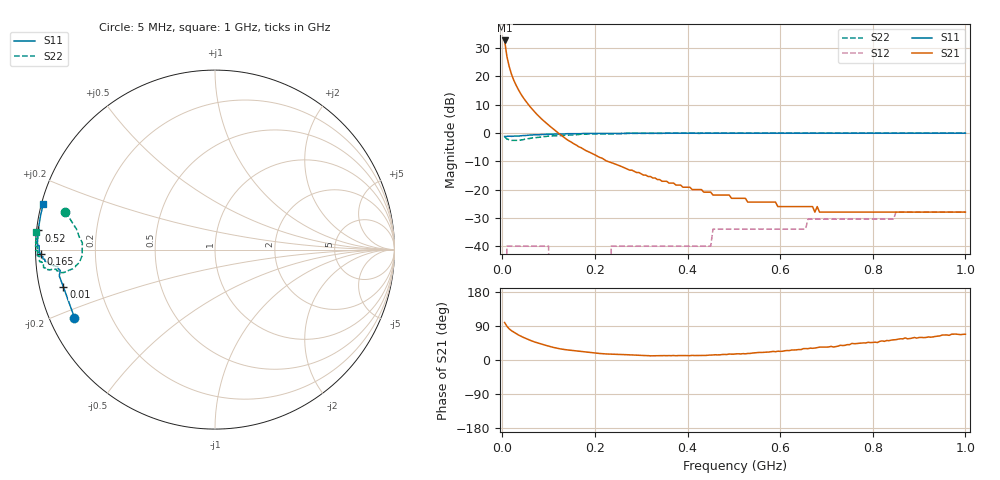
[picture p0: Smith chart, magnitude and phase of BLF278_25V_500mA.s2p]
! Filename:  BLF278_25V_500mA.s2p
! Philips part #: BLF278  !date: 22-05-2003
!Vdd=25V ; Idq=500mA
!D:\Vee measurements\measurement data\VDMOST\BLF278\25V_500mA_#1
# HZ S MA R 50
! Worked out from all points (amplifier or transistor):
!   200 points, 5 MHz to 1 GHz, reference 50 ohm
!   highest |S21| = 32.7 dB at 5 MHz (marker M1)
!   |S21| within 3 dB of that: start of sweep to 7.625 MHz
!   S11 on the Smith chart (normalised r, x): 5 MHz: 0.07, -0.23; 10 MHz: 0.07, -0.12; 165 MHz: 0.02, -0.01; 520 MHz: 0.01, +0.05; 1 GHz: 0.01, +0.13
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5000000  0.87 -154.2  43.03 98.9  0 -7.8  0.86 165.8
1e7  0.87 -166.2  22.29 88.9  0.01 18.0  0.78 171.6
1.5e7  0.88 -170.4  14.8 82.1  0.01 20.1  0.76 174.6
2e7  0.87 -172.3  10.8 77.2  0.01 16.7  0.74 177.1
2.5e7  0.88 -173.1  8.46 73.5  0.01 12.1  0.74 179.5
3e7  0.88 -173.5  6.93 69.6  0.01 6.7  0.74 -179.1
4e7  0.89 -174.0  4.9 62.9  0.01 -1.0  0.75 -175.9
5e7  0.9 -174.3  3.71 57.3  0.01 -7.2  0.78 -173.4
6e7  0.92 -174.7  2.91 52.1  0.01 -12.2  0.8 -172.3
8e7  0.93 -175.5  1.93 43.7  0.01 -18.0  0.84 -171.5
1e8  0.95 -176.3  1.38 36.6  0.01 -18.4  0.88 -171.8
1.05e8  0.95 -176.5  1.27 34.9  0 -17.7  0.88 -172.1
1.65e8  0.97 -178.6  0.57 23.3  0 36.1  0.94 -173.2
1.75e8  0.98 -178.9  0.52 21.9  0 48.2  0.95 -173.5
2.3e8  0.98 179.6  0.31 15.7  0 78.4  0.96 -175.7
2.35e8  0.98 179.4  0.3 15.4  0.01 79.7  0.96 -175.7
3.4e8  0.99 177.3  0.15 11.4  0.01 87.7  0.98 -177.8
5.05e8  0.99 174.1  0.07 16.2  0.02 90.7  0.99 179.8
5.2e8  0.99 173.8  0.07 16.8  0.02 90.8  0.99 179.7
6.7e8  0.99 171.2  0.05 30.9  0.03 91.8  1 177.7
8.35e8  0.99 168.2  0.04 51.0  0.03 94.1  0.99 176.3
1e9  0.99 165.2  0.04 68.0  0.04 93.4  1 174.4
